FUNCTION_BLOCK "Mul_DInt"
VERSION : 0.1
   VAR_INPUT
      "I0.0" : DInt;
      "I0.1" : DInt;
   END_VAR

   VAR_OUTPUT
      "O0.0" : DInt;
   END_VAR


BEGIN
NETWORK
TITLE =
      L #"I0.0";
      L #"I0.1";
      *D;
      T #"O0.0";
      NOP 0;
NETWORK
TITLE =
END_FUNCTION_BLOCK

